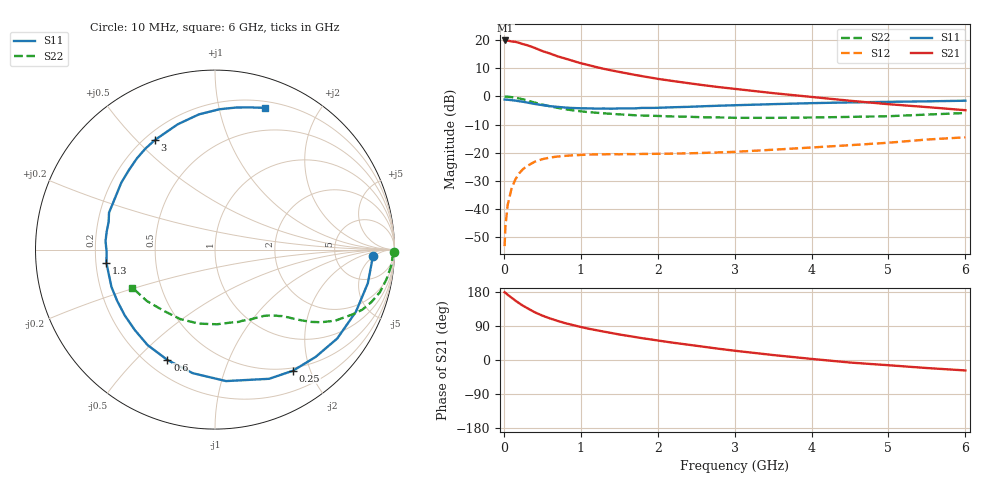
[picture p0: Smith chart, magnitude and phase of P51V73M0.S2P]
! SIEMENS Small Signal Semiconductors
! BFP183
! Si NPN RF Bipolar Junction Transistor in SOT143
! VCE = 1.75 V  IC = 3 mA
! Common Emitter S-Parameters:  March  1996
# GHz  S  MA  R  50
!  f  S11  S21  S12  S22
! GHz  MAG  ANG  MAG  ANG  MAG  ANG  MAG  ANG
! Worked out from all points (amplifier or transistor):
!   36 points, 10 MHz to 6 GHz, reference 50 ohm
!   highest |S21| = 19.8 dB at 20 MHz (marker M1)
!   |S21| within 3 dB of that: start of sweep to 433.4 MHz
!   unconditionally stable (mu >= 1): 1.851 GHz to 5.869 GHz
!   at 250 MHz: K = 0.16, MSG = 22.2 dB, |S12| = -25.8 dB
!   at 1.4 GHz: K = 0.80, MSG = 14.9 dB, |S12| = -20.5 dB
!   at 6 GHz: K = 0.98, MSG = 4.8 dB, |S12| = -14.5 dB
!   S11 on the Smith chart (normalised r, x): 10 MHz: 14, -4; 250 MHz: 0.46, -1.74; 600 MHz: 0.28, -0.62; 1.3 GHz: 0.24, -0.06; 3 GHz: 0.24, +0.57; 6 GHz: 0.26, +1.38
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0.01  0.8798 -2.3  9.694 178.7  0.0022 86.5  0.9959 -0.9
0.02  0.8756 -5.2  9.828 177.4  0.0049 88.3  0.9906 -2.0
0.05  0.8719 -12.4  9.784 172.1  0.0119 85.3  0.9869 -4.9
0.15  0.8421 -36.0  9.282 156.8  0.0337 70.2  0.949 -14.5
0.2  0.8198 -46.8  8.911 149.7  0.0433 65.3  0.9193 -18.5
0.25  0.8026 -57.2  8.45 143.1  0.0513 59.6  0.8863 -22.2
0.3  0.7803 -67.3  8.119 137.4  0.058 55.0  0.8476 -25.2
0.4  0.7351 -85.2  7.265 126.1  0.0691 47.1  0.7781 -30.6
0.5  0.6996 -100.2  6.382 117.2  0.0768 40.7  0.7164 -34.4
0.6  0.6697 -113.3  5.755 109.7  0.0823 35.7  0.6674 -37.1
0.7  0.6512 -125.2  5.136 103.1  0.0857 31.9  0.6259 -39.1
0.8  0.6327 -135.0  4.684 97.1  0.0881 28.7  0.5917 -40.9
0.9  0.6222 -144.0  4.262 92.1  0.0902 26.4  0.5644 -42.3
1.1  0.6132 -160.2  3.592 82.6  0.0927 22.6  0.5256 -44.8
1.3  0.6094 -173.1  3.083 74.9  0.0939 20.0  0.5006 -47.3
1.6  0.6117 170.4  2.561 64.1  0.0947 18.5  0.4723 -51.0
2.2  0.6417 144.4  1.872 45.6  0.0966 18.7  0.4402 -60.6
3  0.6965 118.7  1.361 24.5  0.1038 21.8  0.4167 -76.8
3.5  0.7284 106.6  1.143 13.1  0.1131 23.6  0.4162 -88.5
4.5  0.7822 88.2  0.837 -6.7  0.1362 23.9  0.4328 -116.5
5.5  0.8168 75.9  0.646 -21.2  0.1716 21.3  0.4756 -143.0
6  0.8381 70.4  0.569 -27.6  0.1879 17.7  0.5072 -155.3
